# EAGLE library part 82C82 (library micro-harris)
MICROCONTROLLER/MEMORY DEVICE
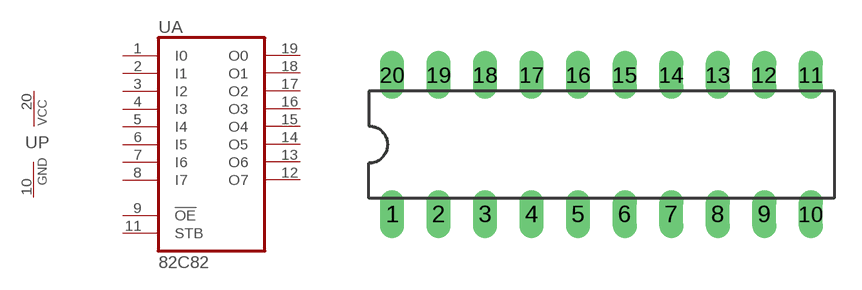
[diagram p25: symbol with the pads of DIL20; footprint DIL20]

Designator prefix U; gates A=82C82 P=PWRN

## 82C82 (MF: INTERSIL; MPN: ID82C82; OC_FARNELL: unknown; OC_NEWARK: 05B7334)  [DIL20]
1  A:I0  in
2  A:I1  in
3  A:I2  in
4  A:I3  in
5  A:I4  in
6  A:I5  in
7  A:I6  in
8  A:I7  in
9  A:!OE  in
10  P:GND  pwr
11  A:STB  in
12  A:O7  out
13  A:O6  out
14  A:O5  out
15  A:O4  out
16  A:O3  out
17  A:O2  out
18  A:O1  out
19  A:O0  out
20  P:VCC  pwr

## Footprint DIL20 (pad centres in mm)
Dual In Line Package
drill 0.813 long: 1 -11.43,-3.81; 2 -8.89,-3.81; 3 -6.35,-3.81; 4 -3.81,-3.81; 5 -1.27,-3.81; 6 1.27,-3.81; 7 3.81,-3.81; 8 6.35,-3.81; 9 8.89,-3.81; 10 11.43,-3.81; 11 11.43,3.81; 12 8.89,3.81; 13 6.35,3.81; 14 3.81,3.81; 15 1.27,3.81; 16 -1.27,3.81; 17 -3.81,3.81; 18 -6.35,3.81; 19 -8.89,3.81; 20 -11.43,3.81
